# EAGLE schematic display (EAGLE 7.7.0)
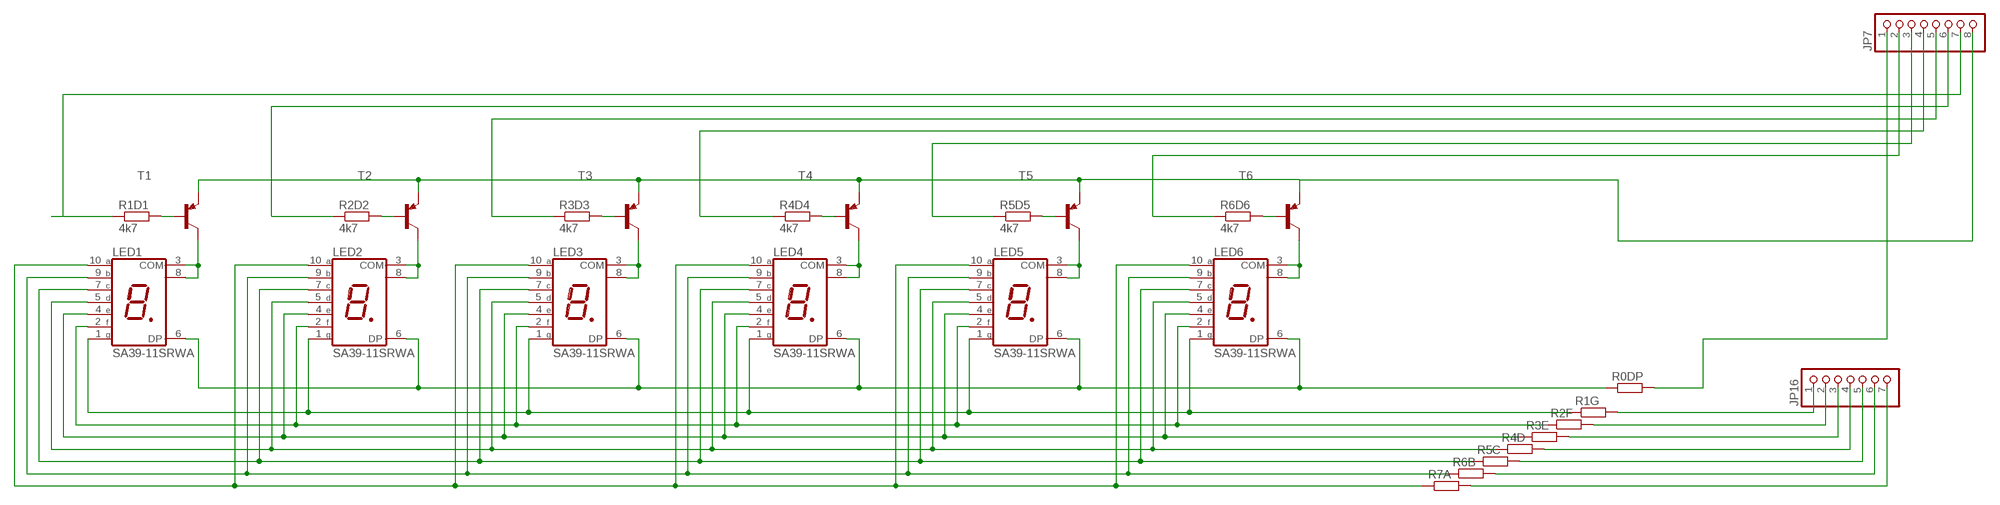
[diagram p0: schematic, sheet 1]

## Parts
JP7  PINHD-1X8  [1X08]
JP16  PINHD-1X7  [1X07]
LED1  SA39-11SRWA  7-SEG_SA39-11SRWA  [SA39-11SRWA]
LED2  SA39-11SRWA  7-SEG_SA39-11SRWA  [SA39-11SRWA]
LED3  SA39-11SRWA  7-SEG_SA39-11SRWA  [SA39-11SRWA]
LED4  SA39-11SRWA  7-SEG_SA39-11SRWA  [SA39-11SRWA]
LED5  SA39-11SRWA  7-SEG_SA39-11SRWA  [SA39-11SRWA]
LED6  SA39-11SRWA  7-SEG_SA39-11SRWA  [SA39-11SRWA]
R0DP  R-EU_M1206  [M1206]
R1D1  4k7  R-EU_M1206  [M1206]
R1G  R-EU_M1206  [M1206]
R2D2  4k7  R-EU_M1206  [M1206]
R2F  R-EU_M1206  [M1206]
R3D3  4k7  R-EU_M1206  [M1206]
R3E  R-EU_M1206  [M1206]
R4D  R-EU_M1206  [M1206]
R4D4  4k7  R-EU_M1206  [M1206]
R5C  R-EU_M1206  [M1206]
R5D5  4k7  R-EU_M1206  [M1206]
R6B  R-EU_M1206  [M1206]
R6D6  4k7  R-EU_M1206  [M1206]
R7A  R-EU_M1206  [M1206]
T1  BC858C-PNP-SOT23-BEC  [SOT23-BEC]
T2  BC858C-PNP-SOT23-BEC  [SOT23-BEC]
T3  BC858C-PNP-SOT23-BEC  [SOT23-BEC]
T4  BC858C-PNP-SOT23-BEC  [SOT23-BEC]
T5  BC858C-PNP-SOT23-BEC  [SOT23-BEC]
T6  BC858C-PNP-SOT23-BEC  [SOT23-BEC]

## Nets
N$1: R1D1.2 T1.B
N$2: R2D2.2 T2.B
N$3: R3D3.2 T3.B
N$4: R4D4.2 T4.B
N$5: R5D5.2 T5.B
N$11: LED1.5(D) LED2.5(D) LED3.5(D) LED4.5(D) LED5.5(D) LED6.5(D) R4D.1
N$16: LED1.3(COM) LED1.8(COM) T1.C
N$17: LED2.3(COM) LED2.8(COM) T2.C
N$19: JP7.4 R4D4.1
N$20: JP7.3 R5D5.1
N$21: JP7.2 R6D6.1
N$25: LED6.3(COM) LED6.8(COM) T6.C
N$26: R6D6.2 T6.B
N$27: LED3.3(COM) LED3.8(COM) T3.C
N$28: JP7.6 R2D2.1
N$31: JP16.2 R2F.2
N$32: JP16.1 R1G.2
N$34: JP7.1 R0DP.2
N$35: LED4.3(COM) LED4.8(COM) T4.C
N$42: JP7.5 R3D3.1
N$44: LED5.3(COM) LED5.8(COM) T5.C
N$52: JP7.8 T1.E T2.E T3.E T4.E T5.E T6.E
N$86: JP7.7 R1D1.1
N$119: LED1.6(DP) LED2.6(DP) LED3.6(DP) LED4.6(DP) LED5.6(DP) LED6.6(DP) R0DP.1
N$121: LED1.7(C) LED2.7(C) LED3.7(C) LED4.7(C) LED5.7(C) LED6.7(C) R5C.1
N$124: LED1.4(E) LED2.4(E) LED3.4(E) LED4.4(E) LED5.4(E) LED6.4(E) R3E.1
N$125: JP16.3 R3E.2
N$128: JP16.5 R5C.2
N$131: JP16.7 R7A.2
N$134: JP16.6 R6B.2
N$168: LED1.10(A) LED2.10(A) LED3.10(A) LED4.10(A) LED5.10(A) LED6.10(A) R7A.1
N$172: LED1.9(B) LED2.9(B) LED3.9(B) LED4.9(B) LED5.9(B) LED6.9(B) R6B.1
N$174: LED1.1(G) LED2.1(G) LED3.1(G) LED4.1(G) LED5.1(G) LED6.1(G) R1G.1
N$175: LED1.2(F) LED2.2(F) LED3.2(F) LED4.2(F) LED5.2(F) LED6.2(F) R2F.1
N$177: JP16.4 R4D.2

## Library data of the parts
JP7 = pinhead:PINHD-1X8: PIN HEADER
JP16 = pinhead:PINHD-1X7: PIN HEADER
LED1-LED6 = display-kingbright:7-SEG_: Kingbright 14.2mm (0.56 INCH) SINGLE DIGIT NUMERIC DUISPLAY Source: SA56-11EWA(Ver1189471036.pdf; OC_FARNELL: unknown; OC_NEWARK: unknown
R0DP R1D1 R1G R2D2 R2F R3D3 R3E R4D R4D4 R5C R5D5 R6B R6D6 R7A = resistor:R-EU_: RESISTOR, European symbol
T1-T6 = transistor:*-PNP-: PNP Transistror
